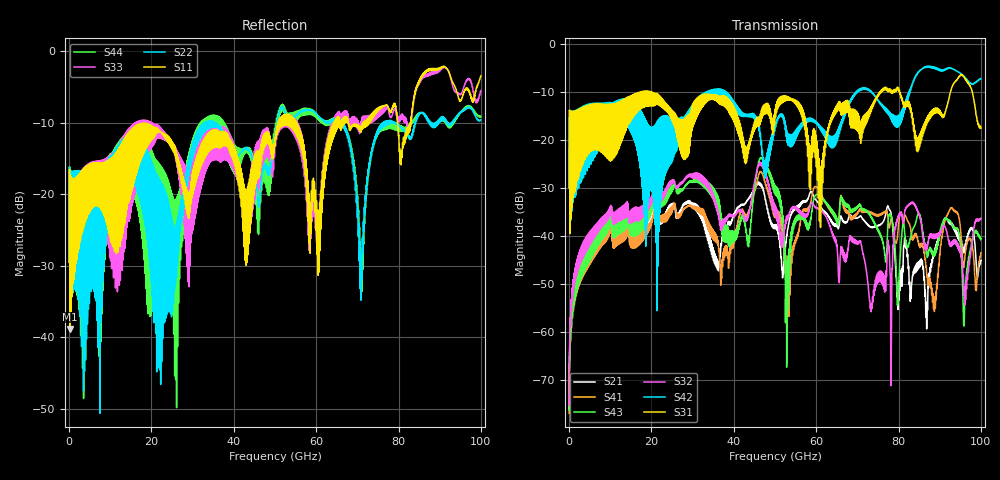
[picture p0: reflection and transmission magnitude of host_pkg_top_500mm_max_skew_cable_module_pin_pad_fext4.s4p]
# Hz S RI R 50
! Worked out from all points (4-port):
!   10000 points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, 10 MHz to 100 GHz, reference 50 ohm
!   strongest paths, dB at 10 MHz, 25.01 GHz, 50.01 GHz, 75.01 GHz, 100 GHz:
!     S31: -29.9, -15.1, -13.5, -10.4, -17.5
!     S42: -29.9, -15.8, -16.8, -11.6, -7.2
!     S32: -75.2, -28.9, -35.1, -49.2, -36.2
!     S43: -76.4, -29.9, -30.1, -38.9, -40.5
!     S41: -76.9, -34.4, -35.4, -35.7, -43.4
!     S21: -76.1, -34.0, -38.4, -37.8, -45.0
!   lowest |S11| = -38.8 dB at 230 MHz (marker M1), VSWR 1.02, Z = 51.1 + j0.262 ohm
!   |S11| at or under -10 dB: start of sweep to 50.81 GHz; 55.14 GHz to 64.4 GHz (9.263 GHz wide, 15.5 % of centre); 67.8 GHz to 71.43 GHz (3.63 GHz wide, 5.21 % of centre)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
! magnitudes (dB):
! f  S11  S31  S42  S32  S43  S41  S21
! 10 MHz  -29.5  -29.9  -29.9  -75.2  -76.4  -76.9  -76.1
! 230 MHz  -38.8  -39.4  -38.8  -57.1  -58.7  -59.6  -58.3
! 9.86 GHz  -24.5  -19.7  -16.6  -33.9  -35.7  -37.2  -36.1
! 46.63 GHz  -13.0  -14.7  -20.6  -25.2  -23.7  -26.7  -29.6
! 52.93 GHz  -9.2  -11.2  -19.9  -36.6  -47.6  -52.8  -39.7
! 73.36 GHz  -9.0  -13.5  -9.8  -55.7  -36.1  -35.2  -38.2
! 100 GHz  -3.5  -17.5  -7.2  -36.2  -40.5  -43.4  -45.0
